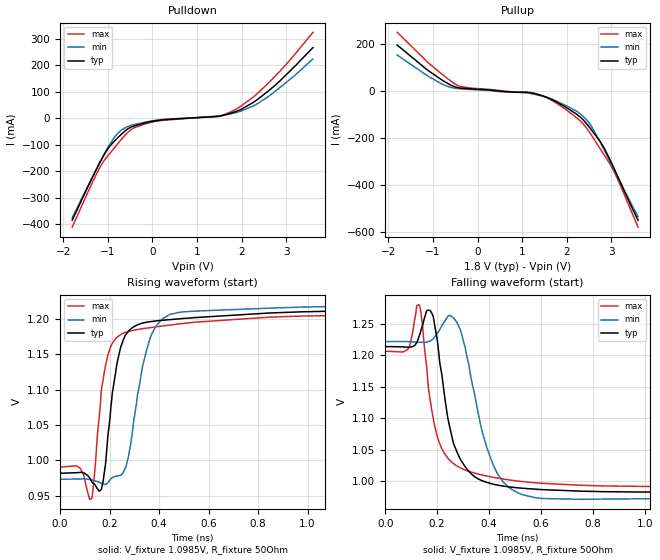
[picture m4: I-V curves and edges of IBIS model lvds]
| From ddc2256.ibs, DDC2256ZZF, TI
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|   lvds Model
[Model]   lvds
Model_type   Output
Polarity   Non-Inverting
Vmeas = 1.0985
Vref = 1.0985
Cref = 2pF
Rref = 50
|   typ   min   max
|   (nom PVT)   (fast PVT)   (slow PVT)
C_comp   3.402e-12   3.166e-12   3.993e-12
| Where nom  PVT is Nominal Process, 1.8V, 27C
|   Fast PVT is Strong Process,  1.9V, 0C
|   Slow PVT is Weak Process,   1.7V, 85C
[Voltage Range]   1.8   1.7   1.9
|Junction Temperature
[Temperature Range]   27   85   0
[Pullup Reference]   1.8   1.7   1.9
[Pulldown Reference]   0   0   0
[Power Clamp Reference]   1.8   1.7   1.9
[GND Clamp Reference]   0   0   0
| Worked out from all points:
|   slope of the pulldown table from 0 to 0.27 V, typ, clamps not added: 44 ohm
|   slope of the pullup table from 0 to 0.27 V, typ, clamps not added: 84.1 ohm
|   falling waveform, V_fixture 1.0985V, R_fixture 50Ohm: 20-80 % time 80.8ps typ, 92.2ps min, 84.5ps max; typ from 1.21 V to 0.982 V
|   rising waveform, V_fixture 1.0985V, R_fixture 50Ohm: 20-80 % time 60.5ps typ, 77ps min, 57.5ps max; typ from 0.982 V to 1.21 V
[Pulldown]
|   Voltage   I(typ)   I(min)   I(max)
-1.8V     -384.7mA   -376.1mA   -411.1mA
-1.168V   -163.5mA   -162.4mA   -182.4mA
-975.4mV  -108.6mA   -103.3mA   -136.4mA
-846mV    -84.78mA   -69.68mA   -110.1mA
-696.1mV  -59.89mA   -44.44mA   -79.42mA
-437.4mV  -30.51mA   -24.83mA   -38.25mA
-76.7mV   -13.96mA   -11.59mA   -17.07mA
1.517V    8.508mA    8.681mA    9.209mA
1.857V    24.74mA    21.06mA    32.67mA
2.265V    60.38mA    46.94mA    80.89mA
2.589V    102mA      81.08mA    131.6mA
3.6V      267mA      224.2mA    324.7mA
[Pullup]
|   Voltage   I(typ)   I(min)   I(max)
-1.8V     194.8mA    152.6mA    249.2mA
-1.114V   88.12mA    63.84mA    121.7mA
-800.4mV  46.84mA    29.55mA    71.63mA
-409.2mV  12.68mA    9.224mA    19.81mA
1.247V    -10.54mA   -12.9mA    -8.085mA
1.66V     -35.98mA   -34.4mA    -39.55mA
2.228V    -99.99mA   -87.29mA   -115.2mA
2.353V    -120mA     -105.5mA   -136.9mA
2.502V    -152.8mA   -136.3mA   -173.1mA
2.768V    -219.8mA   -223.4mA   -251mA
3.075V    -335.1mA   -340.7mA   -348.3mA
3.6V      -549.5mA   -534.1mA   -578.9mA
[Ramp]
R_load = 50
|   typ   min   max
dV/dt_r   0.546627/6.7794e-10   0.437176/1.10982e-09   0.605997/9.93315e-10
dV/dt_f   0.139289/8.07341e-11   0.148795/9.19565e-11   0.129709/8.52113e-11
[Falling Waveform]
V_fixture = 1.0985V
V_fixture_min = 1.0979V
V_fixture_max = 1.0991V
R_fixture = 50Ohm
|   Time   V(typ)   V(min)   V(max)
0s        1.214V     1.221V     1.206V
86.03ps   1.213V     1.222V     1.209V
129.8ps   1.229V     1.221V     1.281V
175ps     1.27V      1.223V     1.124V
212.3ps   1.183V     1.242V     1.057V
276.9ps   1.046V     1.252V     1.024V
369.6ps   1.002V     1.085V     1.01V
433.3ps   993.9mV    1.012V     1.005V
528.2ps   989mV      978.7mV    999.5mV
1.328ns   982mV      973.1mV    990.7mV
[Rising Waveform]
V_fixture = 1.0985V
V_fixture_min = 1.0979V
V_fixture_max = 1.0991V
R_fixture = 50Ohm
|   Time   V(typ)   V(min)   V(max)
0s        981.6mV    973.1mV    990.4mV
81.16ps   982.9mV    973.7mV    988.9mV
127.5ps   970mV      972.4mV    945.7mV
166.6ps   959.3mV    967.3mV    1.099V
182.9ps   993.5mV    965.9mV    1.133V
210.5ps   1.095V     975.5mV    1.165V
253.3ps   1.169V     982mV      1.18V
363.2ps   1.196V     1.173V     1.188V
443.8ps   1.199V     1.206V     1.192V
1.621ns   1.214V     1.221V     1.207V
